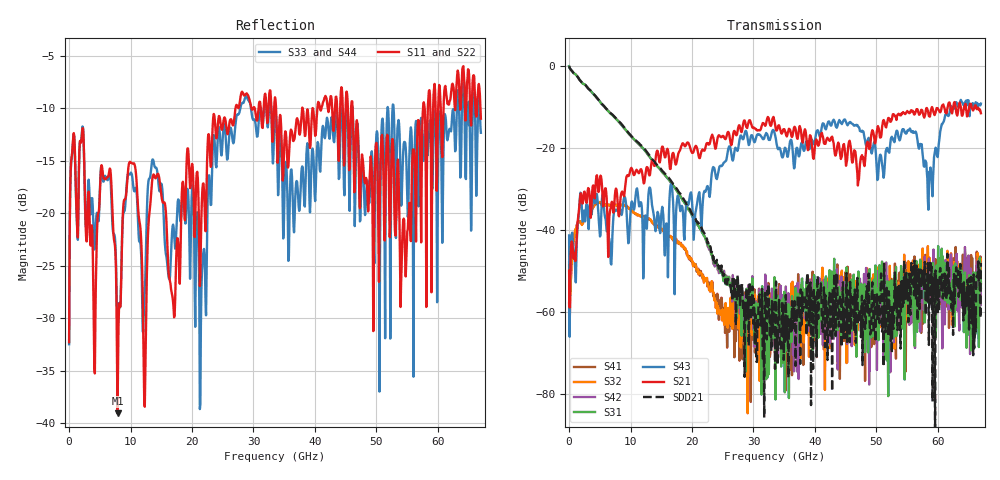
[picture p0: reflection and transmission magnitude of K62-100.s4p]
!Agilent Technologies,N5247A,US50470101,A.10.25.02
!Agilent N5247A: A.10.25.02
!Date: Tuesday, May 12, 2015 13:46:39
!Correction: Sdd11(Full 4 Port(1,2,3,4))
!Sdc11(Full 4 Port(1,2,3,4))
!Sdd12(Full 4 Port(1,2,3,4))
!Sdc12(Full 4 Port(1,2,3,4))
!Scd11(Full 4 Port(1,2,3,4))
!Scc11(Full 4 Port(1,2,3,4))
!Scd12(Full 4 Port(1,2,3,4))
!Scc12(Full 4 Port(1,2,3,4))
!Sdd21(Full 4 Port(1,2,3,4))
!Sdc21(Full 4 Port(1,2,3,4))
!Sdd22(Full 4 Port(1,2,3,4))
!Sdc22(Full 4 Port(1,2,3,4))
!Scd21(Full 4 Port(1,2,3,4))
!Scc21(Full 4 Port(1,2,3,4))
!Scd22(Full 4 Port(1,2,3,4))
!Scc22(Full 4 Port(1,2,3,4))
!Balanced Topology: BBAL
!S4P File: Measurements: <Sdd11,Sdc11,Sdd12,Sdc12>,
!<Scd11,Scc11,Scd12,Scc12>,
!<Sdd21,Sdc21,Sdd22,Sdc22>,
!<Scd21,Scc21,Scd22,Scc22>:
# Hz S  dB  R 50
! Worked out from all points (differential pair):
!   801 points, 10 MHz to 67 GHz, reference 50 ohm
!   strongest paths, dB at 10 MHz, 16.76 GHz, 33.51 GHz, 50.25 GHz, 67 GHz:
!     S21: -49.9, -21.9, -14.2, -14.7, -11.6
!     S43: -41.3, -29.6, -16.8, -27.6, -9.2
!     S31: -0.1, -28.8, -60.3, -54.3, -54.1
!     S42: -0.1, -28.8, -60.6, -50.0, -52.7
!     S32: -47.9, -41.8, -58.3, -57.8, -47.1
!     S41: -57.7, -42.1, -69.9, -55.9, -53.0
!   taken as a pair (ports 1,2 in; 3,4 out), SDD21 dB: -0.1, -28.4, -73.8, -59.1, -48.0
!   lowest |S11| = -39.1 dB at 7.881 GHz (marker M1), VSWR 1.02, Z = 49.6 - j1.03 ohm
!   |S11| at or under -10 dB: start of sweep to 27.07 GHz; 33.68 GHz to 37.93 GHz (4.251 GHz wide, 11.9 % of centre); 46.13 GHz to 57.59 GHz (11.46 GHz wide, 22.1 % of centre)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
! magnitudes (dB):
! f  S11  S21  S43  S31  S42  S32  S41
! 10 MHz  -32.3  -49.9  -41.3  -0.1  -0.1  -47.9  -57.7
! 2.02 GHz  -13.0  -31.7  -32.6  -3.9  -3.9  -38.5  -38.4
! 7.881 GHz  -39.1  -32.8  -35.0  -13.3  -13.3  -34.1  -33.9
! 32.42 GHz  -10.4  -12.6  -17.8  -56.4  -61.6  -55.5  -52.9
! 47.07 GHz  -13.8  -28.1  -14.9  -50.1  -56.6  -56.2  -54.7
! 58.71 GHz  -8.7  -12.4  -26.4  -51.2  -48.3  -52.3  -52.5
! 67 GHz  -11.0  -11.6  -9.2  -54.1  -52.7  -47.1  -53.0
